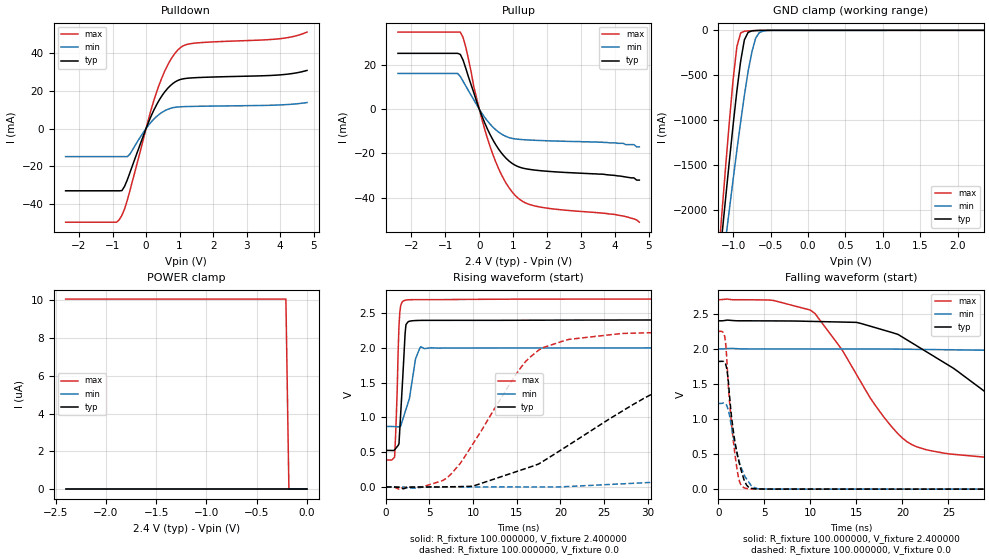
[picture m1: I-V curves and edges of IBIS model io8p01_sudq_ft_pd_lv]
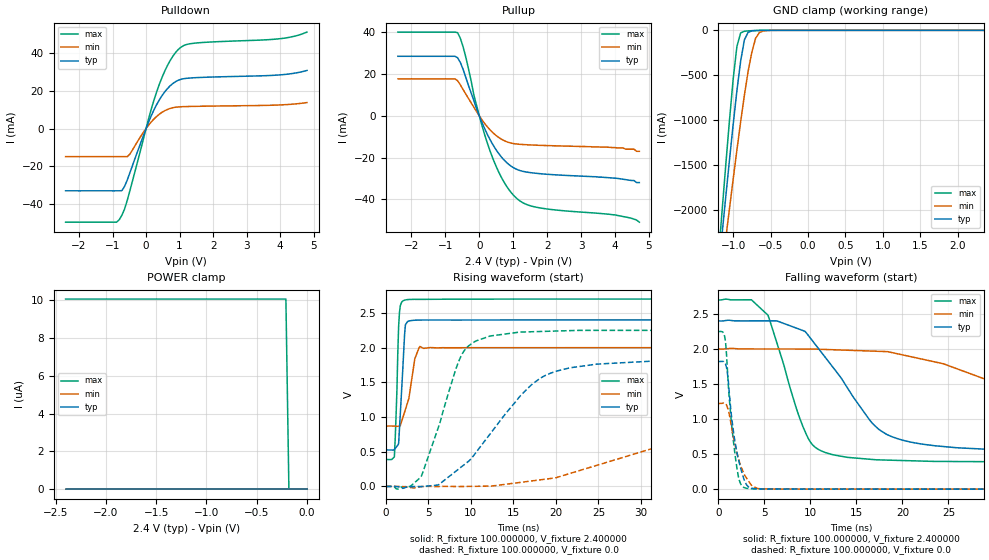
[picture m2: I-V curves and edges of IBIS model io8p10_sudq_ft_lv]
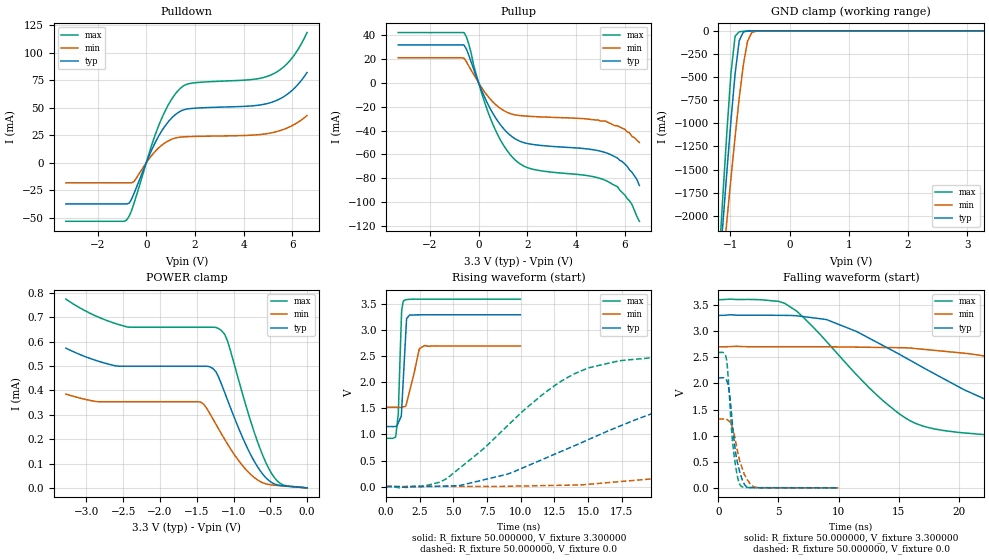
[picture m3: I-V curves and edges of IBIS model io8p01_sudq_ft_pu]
|   stm32f0_440_ufbga64 IBIS Model
[IBIS ver]   4.2
[File name]  stm32f0_440_ufbga64.ibs
[File Rev]   1.0
[Date]   15-5-2013
[Source] Data Created at STMicroelectronics
[Notes]   File originated from ELDO simulations.
[Disclaimer]  This information is for modeling purpose only and is
   not guaranted. The information is subject to change without
   notice.
[Copyright] Copyright 2015 STMicroelectronics Inc.
[Component] stm32f0_440_ufbga64
[Manufacturer] STMicroelectronics
[Package]
| variable   typ   min   max
R_pkg   0.0   NA   NA
L_pkg   0.0H   NA   NA
C_pkg   0.0F   NA   NA
[Pin] signal_name  model_name   R_pin   L_pin   C_pin
B2   VBAT  POWER
A2   PC13  io8p_sudq_tc
A1   PC14  io8p_sudq_tc
B1   PC15  io8p_sudq_tc
C1   PF0   io8p_sudq_ft
D1   PF1   io8p_sudq_ft
E1   NRST  ioreset_tc_v33
E3   PC0   io8p_sudq_ft
E2   PC1   io8p_sudq_ft
F2   PC2   io8p_sudq_ft
G1   PC3   io8p_sudq_ft
F1   VSSA  GND
H1   VDDA  POWER
G2   PA0   io8p_sudq_ft
H2   PA1   io8p_sudq_ft
F3   PA2   io8p_sudq_ft
G3   PA3   io8p_sudq_ft
C2   PF4   io8p_sudq_ft
D2   PF5   io8p_sudq_ft
H3   PA4   io8p_sudq_ft
F4   PA5   io8p_sudq_ft
G4   PA6   io8p_sudq_ft
H4   PA7   io8p_sudq_ft
H5   PC4   io8p_sudq_ft
H6   PC5   io8p_sudq_ft
F5   PB0   io8p_sudq_ft
G5   PB1   io8p_sudq_ft
G6   PB2   io8p_sudq_ft
G7   PB10  io8p_sudq_i2cin_lv_ft
H7   PB11  io8p_sudq_i2cin_lv_ft
D4   VSS   GND
E4   VDD   POWER
H8   PB12  io8p_sudq_ft
G8   PB13  io8p_sudq_ft
F8   PB14  io8p_sudq_ft
F7   PB15  io8p_sudq_ft
F6   PC6   io8p_sudq_ft
E7   PC7   io8p_sudq_ft
E8   PC8   io8p_sudq_ft
D8   PC9   io8p_sudq_ft
D7   PA8   io8p_sudq_ft
C7   PA9   io8p_sudq_ft
C6   PA10  io8p_sudq_ft
C8   PA11  io8p_sudq_ft
B8   PA12  io8p_sudq_ft
A8   PA13  io8p_sudq_ft
D6   PF6   io8p_sudq_i2cin_lv_ft
E6   PF7   io8p_sudq_i2cin_lv_ft
A7   PA14  io8p_sudq_ft
A6   PA15  io8p_sudq_ft
B7   PC10  io8p_sudq_ft
B6   PC11  io8p_sudq_ft
C5   PC12  io8p_sudq_ft
B5   PD2   io8p_sudq_ft
A5   PB3   io8p_sudq_ft
A4   PB4   io8p_sudq_ft
C4   PB5   io8p_sudq_ft
D3   PB6   io8p_sudq_i2cin_lv_ft
C3   PB7   io8p_sudq_i2cin_lv_ft
B4   BOOT0 vpp_test_hv
B3   PB8   io8p_sudq_i2cin_lv_ft
A3   PB9   io8p_sudq_i2cin_lv_ft
D5   VSS   GND
E5   VDD   POWER
[Model Selector] io8p_sudq_ft
io8p01_sudq_ft_pd_lv  "SPEED01 2P0V, PD=40kOhm"
io8p01_sudq_ft_pu_lv  "SPEED01 2P0V, PU=40kOhm"
io8p01_sudq_ft_lv  "SPEED01 2P0V"
io8p10_sudq_ft_pd_lv  "SPEED10 2P0V, PD=40kOhm"
io8p10_sudq_ft_pu_lv  "SPEED10 2P0V, PU=40kOhm"
io8p10_sudq_ft_lv  "SPEED10 2P0V"
io8p11_sudq_ft_pd_lv  "SPEED11 2P0V, PD=40kOhm"
io8p11_sudq_ft_pu_lv  "SPEED11 2P0V, PU=40kOhm"
io8p11_sudq_ft_lv  "SPEED11 2P0V"
io8p01_sudq_ft_pd  "SPEED01, PD=40kOhm"
io8p01_sudq_ft_pu  "SPEED01, PU=40kOhm"
io8p01_sudq_ft  "SPEED01"
io8p10_sudq_ft_pd  "SPEED10, PD=40kOhm"
io8p10_sudq_ft_pu  "SPEED10, PU=40kOhm"
io8p10_sudq_ft  "SPEED10"
io8p11_sudq_ft_pd  "SPEED11, PD=40kOhm"
io8p11_sudq_ft_pu  "SPEED11, PU=40kOhm"
io8p11_sudq_ft  "SPEED11"
[Model Selector] io8p_sudq_i2cin_lv_ft
io8p01_sudq_i2cin_lv_ft_pd_lv  "SPEED01 2P0V, PD=40kOhm"
io8p01_sudq_i2cin_lv_ft_pu_lv  "SPEED01 2P0V, PU=40kOhm"
io8p01_sudq_i2cin_lv_ft_lv  "SPEED01 2P0V"
io8p10_sudq_i2cin_lv_ft_pd_lv  "SPEED10 2P0V, PD=40kOhm"
io8p10_sudq_i2cin_lv_ft_pu_lv  "SPEED10 2P0V, PU=40kOhm"
io8p10_sudq_i2cin_lv_ft_lv  "SPEED10 2P0V"
io8p11_sudq_i2cin_lv_ft_pd_lv  "SPEED11 2P0V, PD=40kOhm"
io8p11_sudq_i2cin_lv_ft_pu_lv  "SPEED11 2P0V, PU=40kOhm"
io8p11_sudq_i2cin_lv_ft_lv  "SPEED11 2P0V"
io8p01_sudq_i2cin_lv_ft_pd  "SPEED01, PD=40kOhm"
io8p01_sudq_i2cin_lv_ft_pu  "SPEED01, PU=40kOhm"
io8p01_sudq_i2cin_lv_ft  "SPEED01"
io8p10_sudq_i2cin_lv_ft_pd  "SPEED10, PD=40kOhm"
io8p10_sudq_i2cin_lv_ft_pu  "SPEED10, PU=40kOhm"
io8p10_sudq_i2cin_lv_ft  "SPEED10"
io8p11_sudq_i2cin_lv_ft_pd  "SPEED11, PD=40kOhm"
io8p11_sudq_i2cin_lv_ft_pu  "SPEED11, PU=40kOhm"
io8p11_sudq_i2cin_lv_ft  "SPEED11"
[Model Selector] io8p_sudq_tc
io8p01_sudq_tc_pd_lv  "SPEED01 2P0V, PD=40kOhm"
io8p01_sudq_tc_pu_lv  "SPEED01 2P0V, PU=40kOhm"
io8p01_sudq_tc_lv  "SPEED01 2P0V"
io8p10_sudq_tc_pd_lv  "SPEED10 2P0V, PD=40kOhm"
io8p10_sudq_tc_pu_lv  "SPEED10 2P0V, PU=40kOhm"
io8p10_sudq_tc_lv  "SPEED10 2P0V"
io8p11_sudq_tc_pd_lv  "SPEED11 2P0V, PD=40kOhm"
io8p11_sudq_tc_pu_lv  "SPEED11 2P0V, PU=40kOhm"
io8p11_sudq_tc_lv  "SPEED11 2P0V"
io8p01_sudq_tc_pd  "SPEED01, PD=40kOhm"
io8p01_sudq_tc_pu  "SPEED01, PU=40kOhm"
io8p01_sudq_tc  "SPEED01"
io8p10_sudq_tc_pd  "SPEED10, PD=40kOhm"
io8p10_sudq_tc_pu  "SPEED10, PU=40kOhm"
io8p10_sudq_tc  "SPEED10"
io8p11_sudq_tc_pd  "SPEED11, PD=40kOhm"
io8p11_sudq_tc_pu  "SPEED11, PU=40kOhm"
io8p11_sudq_tc  "SPEED11"
[Model Selector] ioreset_tc_v33
ioreset_tc_v33_pu_lv  "IORESET 2V + PU=40kOhm"
ioreset_tc_v33_nopu_lv  "IORESET 2V"
ioreset_tc_v33_pu  "IORESET + PU=40kOhm"
ioreset_tc_v33_nopu  "IORESET"
[Model Selector] vpp_test_hv
vpp_test_hv_3p3  "Input Buffer"
vpp_test_hv_2p4  "Input Buffer 2P0V"
| Models and submodels in the file (60): io8p01_sudq_ft_pd_lv (I/O), io8p01_sudq_ft_pu_lv (I/O), io8p01_sudq_ft_lv (I/O), io8p10_sudq_ft_pd_lv (I/O), io8p10_sudq_ft_pu_lv (I/O), io8p10_sudq_ft_lv (I/O), io8p11_sudq_ft_pd_lv (I/O), io8p11_sudq_ft_pu_lv (I/O), io8p11_sudq_ft_lv (I/O), io8p01_sudq_ft_pd (I/O), io8p01_sudq_ft_pu (I/O), io8p01_sudq_ft (I/O), io8p10_sudq_ft_pd (I/O), io8p10_sudq_ft_pu (I/O), io8p10_sudq_ft (I/O), io8p11_sudq_ft_pd (I/O), io8p11_sudq_ft_pu (I/O), io8p11_sudq_ft (I/O), io8p01_sudq_i2cin_lv_ft_pd_lv (I/O), io8p01_sudq_i2cin_lv_ft_pu_lv (I/O), io8p01_sudq_i2cin_lv_ft_lv (I/O), io8p10_sudq_i2cin_lv_ft_pd_lv (I/O), io8p10_sudq_i2cin_lv_ft_pu_lv (I/O), io8p10_sudq_i2cin_lv_ft_lv (I/O), io8p11_sudq_i2cin_lv_ft_pd_lv (I/O), io8p11_sudq_i2cin_lv_ft_pu_lv (I/O), io8p11_sudq_i2cin_lv_ft_lv (I/O), io8p01_sudq_i2cin_lv_ft_pd (I/O), io8p01_sudq_i2cin_lv_ft_pu (I/O), io8p01_sudq_i2cin_lv_ft (I/O), io8p10_sudq_i2cin_lv_ft_pd (I/O), io8p10_sudq_i2cin_lv_ft_pu (I/O), io8p10_sudq_i2cin_lv_ft (I/O), io8p11_sudq_i2cin_lv_ft_pd (I/O), io8p11_sudq_i2cin_lv_ft_pu (I/O), io8p11_sudq_i2cin_lv_ft (I/O), io8p01_sudq_tc_pd_lv (I/O), io8p01_sudq_tc_pu_lv (I/O), io8p01_sudq_tc_lv (I/O), io8p10_sudq_tc_pd_lv (I/O), io8p10_sudq_tc_pu_lv (I/O), io8p10_sudq_tc_lv (I/O), io8p11_sudq_tc_pd_lv (I/O), io8p11_sudq_tc_pu_lv (I/O), io8p11_sudq_tc_lv (I/O), io8p01_sudq_tc_pd (I/O), io8p01_sudq_tc_pu (I/O), io8p01_sudq_tc (I/O), io8p10_sudq_tc_pd (I/O), io8p10_sudq_tc_pu (I/O), io8p10_sudq_tc (I/O), io8p11_sudq_tc_pd (I/O), io8p11_sudq_tc_pu (I/O), io8p11_sudq_tc (I/O), ioreset_tc_v33_pu_lv (I/O_open_drain), ioreset_tc_v33_nopu_lv (I/O_open_drain), ioreset_tc_v33_pu (I/O_open_drain), ioreset_tc_v33_nopu (I/O_open_drain), vpp_test_hv_2p4 (Input), vpp_test_hv_3p3 (Input)
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|   Model io8p01_sudq_ft_pd_lv
[Model]  io8p01_sudq_ft_pd_lv
Model_type I/O
Polarity   Non-Inverting
Enable   Active-Low
Vinl =   0.720000V
Vinh =   1.680000V
Vmeas =  1.200000V
Cref =   50.000000pF
Rref =   100.000000M
Vref =   0.0V
C_comp   1.970100pF   1.887900pF   2.069400pF
[Temperature Range]   25.000000   0.125000k   -40.000000
[Pullup Reference]   2.400000V   2.000000V   2.700000V
[Pulldown Reference]   0.0V   0.0V   0.0V
[POWER Clamp Reference]   2.400000V   2.000000V   2.700000V
[GND Clamp Reference]   0.0V   0.0V   0.0V
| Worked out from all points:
|   slope of the pulldown table from 0 to 0.36 V, typ, clamps not added: 25.5 ohm
|   slope of the pullup table from 0 to 0.36 V, typ, clamps not added: 28.4 ohm
|   GND clamp passes 1 mA (typ) near -0.64 V on its own axis
|   rising waveform, R_fixture 100.000000, V_fixture 2.400000: 20-80 % time 499ps typ, 1.06ns min, 336ps max; typ from 0.525 V to 2.4 V
|   rising waveform, R_fixture 100.000000, V_fixture 0.0: 20-80 % time 14.6ns typ, 43.7ns min, 6.88ns max; typ from 0 V to 1.82 V
|   falling waveform, R_fixture 100.000000, V_fixture 2.400000: 20-80 % time 12.9ns typ, 32.5ns min, 7.07ns max; typ from 2.4 V to 0.525 V
|   falling waveform, R_fixture 100.000000, V_fixture 0.0: 20-80 % time 1.15ns typ, 1.36ns min, 910ps max; typ from 1.82 V to 0 V
[Pulldown]
|Voltage   I(typ)   I(min)   I(max)
-2.4V     -33.16mA   -14.98mA   -49.86mA
-880mV    -33.16mA   -14.98mA   -49.86mA
-800mV    -33.16mA   -14.98mA   -48.55mA
-640mV    -30.75mA   -14.98mA   -42.76mA
-480mV    -23.43mA   -13.57mA   -32.92mA
80mV      3.651mA    1.905mA    5.506mA
400mV     15.37mA    7.665mA    23.73mA
720mV     22.75mA    10.69mA    36.23mA
1.04V     26.18mA    11.57mA    43.27mA
1.52V     27.09mA    11.81mA    45.55mA
4V        28.55mA    12.55mA    47.81mA
4.8V      30.9mA     13.81mA    51.31mA
[Pullup]
|Voltage   I(typ)   I(min)   I(max)
-2.4V     25.2mA     16.13mA    34.79mA
-640mV    25.2mA     16.13mA    34.79mA
-560mV    24.71mA    14.75mA    34.79mA
-400mV    18.51mA    10.48mA    28.09mA
-160mV    7.338mA    4.152mA    10.02mA
80mV      -3.229mA   -1.94mA    -4.736mA
400mV     -13.82mA   -8.081mA   -20.45mA
800mV     -22.31mA   -12.38mA   -33.66mA
1.2V      -26.24mA   -13.65mA   -40.83mA
1.76V     -27.69mA   -14.12mA   -44.07mA
4V        -29.9mA    -15.2mA    -47.5mA
4.72V     -32mA      -17mA      -51mA
[GND_clamp]
|Voltage   I(typ)   I(min)   I(max)
-2.4V     -9.788A    -9.782A    -9.734A
-1.2V     -2.718A    -3.021A    -2.568A
-1.15V    -2.29A     -2.675A    -2.036A
-1.1V     -1.868A    -2.333A    -1.515A
-1.05V    -1.454A    -1.995A    -1.012A
-950mV    -674.5mA   -1.337A    -180.6mA
-900mV    -345.2mA   -1.023A    -29.74mA
-850mV    -106.4mA   -726mA     -10.14mA
-750mV    -6.411mA   -244mA     -4.042mA
-700mV    -2.572mA   -88.62mA   -2.346mA
-600mV    -429.6uA   -7.75mA    -383.5uA
2.35V     59.77uA    46.33uA    66.89uA
[POWER_clamp]
|Voltage   I(typ)   I(min)   I(max)
-2.4V     0A         0A         10.06uA
-210mV    0A         0A         10.06uA
-180mV    0A         0A         0A
0V        0A         0A         0A
[Ramp]
| variable   typ   min   max
dV/dt_r  1.09218/14.55718n   0.73266/43.64565n   1.34874/6.87247n
dV/dt_f  1.12429/12.86053n   0.67801/32.45722n   1.38701/7.06387n
R_load = 100.000000
[Rising Waveform]
R_fixture= 100.000000
V_fixture= 2.400000
V_fixture_min= 2.000000
V_fixture_max= 2.700000
|time   V(typ)   V(min)   V(max)
0s        524.8mV    868.7mV    387.2mV
1.001ns   533mV      867mV      427.7mV
1.301ns   579.7mV    865.4mV    1.395V
1.502ns   618.4mV    864.7mV    2.307V
1.602ns   837.8mV    864.4mV    2.512V
2.102ns   1.961V     1.034V     2.677V
2.302ns   2.331V     1.113V     2.684V
3.403ns   2.39V      1.843V     2.691V
4.004ns   2.392V     2.014V     2.691V
49.85ns   2.399V     1.999V     2.699V
[Rising Waveform]
R_fixture= 100.000000
V_fixture= 0.0
V_fixture_min= 0.0
V_fixture_max= 0.0
|time   V(typ)   V(min)   V(max)
0s        1.768nV    15.89nV    1.355nV
7.007ns   1.867mV    822uV      130.1mV
15.02ns   222.8mV    610.6uV    1.635V
17.52ns   330.7mV    351.7uV    1.966V
27.03ns   1.085V     44.44mV    2.204V
34.53ns   1.55V      90.81mV    2.229V
43.04ns   1.723V     239mV      2.246V
84.08ns   1.82V      945.5mV    2.248V
103.1ns   1.82V      1.111V     2.248V
249.2ns   1.82V      1.221V     2.248V
[Falling Waveform]
R_fixture= 100.000000
V_fixture= 2.400000
V_fixture_min= 2.000000
V_fixture_max= 2.700000
|time   V(typ)   V(min)   V(max)
0s        2.399V     1.999V     2.699V
10.01ns   2.391V     1.998V     2.551V
15.02ns   2.376V     1.997V     1.633V
20.02ns   2.165V     1.994V     725.2mV
29.53ns   1.332V     1.979V     449.6mV
35.04ns   877.6mV    1.964V     425.1mV
42.54ns   673.2mV    1.851V     405.8mV
67.07ns   552.7mV    1.286V     389.2mV
85.59ns   536.1mV    1.035V     387.2mV
249.2ns   524.8mV    868.7mV    387.2mV
[Falling Waveform]
R_fixture= 100.000000
V_fixture= 0.0
V_fixture_min= 0.0
V_fixture_max= 0.0
|time   V(typ)   V(min)   V(max)
0s        1.82V      1.221V     2.248V
700.7ps   1.801V     1.221V     2.178V
800.8ps   1.783V     1.214V     2.095V
1.001ns   1.652V     1.164V     1.701V
1.401ns   1.088V     921.6mV    989mV
1.802ns   687.3mV    646.2mV    513.2mV
2.302ns   364.2mV    381.5mV    115.5mV
2.903ns   104.2mV    178.7mV    14.94mV
4.705ns   1.559mV    3.204mV    789.6uV
49.85ns   1.768nV    15.89nV    1.355nV
|   Model io8p10_sudq_ft_lv
[Model]  io8p10_sudq_ft_lv
Model_type I/O
Polarity   Non-Inverting
Enable   Active-Low
Vinl =   0.720000V
Vinh =   1.680000V
Vmeas =  1.200000V
Cref =   50.000000pF
Rref =   100.000000M
Vref =   0.0V
C_comp   1.970100pF   1.887900pF   2.069400pF
[Temperature Range]   25.000000   0.125000k   -40.000000
[Pullup Reference]   2.400000V   2.000000V   2.700000V
[Pulldown Reference]   0.0V   0.0V   0.0V
[POWER Clamp Reference]   2.400000V   2.000000V   2.700000V
[GND Clamp Reference]   0.0V   0.0V   0.0V
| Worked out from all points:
|   slope of the pulldown table from 0 to 0.36 V, typ, clamps not added: 25.5 ohm
|   slope of the pullup table from 0 to 0.36 V, typ, clamps not added: 28.4 ohm
|   GND clamp passes 1 mA (typ) near -0.64 V on its own axis
|   rising waveform, R_fixture 100.000000, V_fixture 2.400000: 20-80 % time 501ps typ, 1.06ns min, 336ps max; typ from 0.525 V to 2.4 V
|   rising waveform, R_fixture 100.000000, V_fixture 0.0: 20-80 % time 7.32ns typ, 21.7ns min, 3.52ns max; typ from 0 V to 1.82 V
|   falling waveform, R_fixture 100.000000, V_fixture 2.400000: 20-80 % time 6.27ns typ, 18.5ns min, 3.33ns max; typ from 2.4 V to 0.525 V
|   falling waveform, R_fixture 100.000000, V_fixture 0.0: 20-80 % time 1.16ns typ, 1.4ns min, 914ps max; typ from 1.82 V to 0 V
[Pulldown]
|Voltage   I(typ)   I(min)   I(max)
-2.4V     -33.16mA   -14.98mA   -49.86mA
-880mV    -33.16mA   -14.98mA   -49.86mA
-800mV    -33.16mA   -14.98mA   -48.55mA
-640mV    -30.75mA   -14.98mA   -42.76mA
-480mV    -23.43mA   -13.57mA   -32.92mA
80mV      3.651mA    1.905mA    5.506mA
400mV     15.37mA    7.665mA    23.73mA
720mV     22.75mA    10.69mA    36.23mA
1.04V     26.18mA    11.57mA    43.27mA
1.52V     27.09mA    11.81mA    45.55mA
4V        28.55mA    12.55mA    47.81mA
4.8V      30.9mA     13.81mA    51.31mA
[Pullup]
|Voltage   I(typ)   I(min)   I(max)
-2.4V     28.57mA    17.75mA    40.17mA
-720mV    28.57mA    17.75mA    40.17mA
-640mV    27.85mA    16.83mA    39.88mA
-480mV    22.38mA    12.65mA    33.22mA
-80mV     3.427mA    2.066mA    4.957mA
160mV     -6.219mA   -3.715mA   -9.137mA
320mV     -11.51mA   -6.781mA   -16.98mA
720mV     -21mA      -11.8mA    -31.54mA
1.12V     -25.77mA   -13.54mA   -39.82mA
1.76V     -27.69mA   -14.12mA   -44.07mA
4V        -29.9mA    -15.2mA    -47.5mA
4.72V     -32mA      -17mA      -51mA
[GND_clamp]
|Voltage   I(typ)   I(min)   I(max)
-2.4V     -9.788A    -9.782A    -9.734A
-1.2V     -2.718A    -3.02A     -2.568A
-1.15V    -2.29A     -2.675A    -2.036A
-1.1V     -1.868A    -2.333A    -1.515A
-1.05V    -1.454A    -1.995A    -1.012A
-950mV    -674.5mA   -1.337A    -180.5mA
-900mV    -345.2mA   -1.023A    -29.72mA
-850mV    -106.4mA   -726mA     -10.13mA
-750mV    -6.396mA   -244mA     -4.026mA
-700mV    -2.558mA   -88.61mA   -2.329mA
-600mV    -416uA     -7.739mA   -368uA
2.35V     0A         0A         0A
[POWER_clamp]
|Voltage   I(typ)   I(min)   I(max)
-2.4V     0A         0A         10.06uA
-210mV    0A         0A         10.06uA
-180mV    0A         0A         0A
0V        0A         0A         0A
[Ramp]
| variable   typ   min   max
dV/dt_r  1.09308/7.31082n   0.73308/21.71145n   1.34964/3.51759n
dV/dt_f  1.12481/6.26349n   0.67631/18.49686n   1.38754/3.32485n
R_load = 100.000000
[Rising Waveform]
R_fixture= 100.000000
V_fixture= 2.400000
V_fixture_min= 2.000000
V_fixture_max= 2.700000
|time   V(typ)   V(min)   V(max)
0s        525.2mV    870.3mV    387.4mV
1.001ns   533.2mV    868.7mV    426.9mV
1.301ns   579.1mV    867.1mV    1.388V
1.502ns   617.1mV    866.5mV    2.304V
1.702ns   1.054V     877mV      2.604V
2.202ns   2.189V     1.072V     2.684V
2.603ns   2.379V     1.227V     2.693V
3.403ns   2.395V     1.838V     2.696V
4.004ns   2.397V     2.017V     2.696V
49.85ns   2.4V       2V         2.7V
[Rising Waveform]
R_fixture= 100.000000
V_fixture= 0.0
V_fixture_min= 0.0
V_fixture_max= 0.0
|time   V(typ)   V(min)   V(max)
0s        1.81nV     16.19nV    1.388nV
2.803ns   -3.281mV   -14.07mV   -1.578mV
4.204ns   -1.834mV   -2.504mV   153.3mV
8.809ns   274.6mV    -1.375mV   1.87V
12.21ns   748.9mV    4.656mV    2.166V
18.02ns   1.547V     92.84mV    2.232V
24.82ns   1.763V     304.5mV    2.249V
40.24ns   1.817V     861.6mV    2.249V
51.85ns   1.822V     1.107V     2.249V
99.7ns    1.822V     1.223V     2.249V
[Falling Waveform]
R_fixture= 100.000000
V_fixture= 2.400000
V_fixture_min= 2.000000
V_fixture_max= 2.700000
|time   V(typ)   V(min)   V(max)
0s        2.4V       2V         2.7V
3.604ns   2.401V     2V         2.703V
5.405ns   2.402V     2V         2.482V
9.81ns    2.189V     2V         715.2mV
14.01ns   1.448V     1.982V     453.6mV
18.22ns   786.7mV    1.963V     414.6mV
25.83ns   591.3mV    1.722V     393.9mV
36.04ns   545.2mV    1.277V     387.5mV
53.05ns   528.1mV    942.3mV    387.4mV
99.7ns    525.2mV    870.3mV    387.4mV
[Falling Waveform]
R_fixture= 100.000000
V_fixture= 0.0
V_fixture_min= 0.0
V_fixture_max= 0.0
|time   V(typ)   V(min)   V(max)
0s        1.822V     1.223V     2.249V
700.7ps   1.802V     1.222V     2.18V
800.8ps   1.785V     1.215V     2.098V
1.001ns   1.656V     1.165V     1.707V
1.401ns   1.093V     924.2mV    997.1mV
1.902ns   616.8mV    592mV      421.8mV
2.302ns   368.5mV    388.7mV    122.4mV
2.903ns   107.4mV    191.2mV    17.72mV
4.705ns   2.748mV    4.47mV     1.93mV
49.85ns   1.81nV     16.19nV    1.388nV
|   Model io8p01_sudq_ft_pu
[Model]  io8p01_sudq_ft_pu
Model_type I/O
Polarity   Non-Inverting
Enable   Active-Low
Vinl =   0.990000V
Vinh =   2.310000V
Vmeas =  1.650000V
Cref =   50.000000pF
Rref =   100.000000M
Vref =   0.0V
C_comp   1.970900pF   1.892300pF   2.063200pF
[Temperature Range]   25.000000   0.125000k   -40.000000
[Pullup Reference]   3.300000V   2.700000V   3.600000V
[Pulldown Reference]   0.0V   0.0V   0.0V
[POWER Clamp Reference]   3.300000V   2.700000V   3.600000V
[GND Clamp Reference]   0.0V   0.0V   0.0V
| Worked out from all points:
|   slope of the pulldown table from 0 to 0.495 V, typ, clamps not added: 20.9 ohm
|   slope of the pullup table from 0 to 0.495 V, typ, clamps not added: 22.2 ohm
|   GND clamp passes 1 mA (typ) near -0.64 V on its own axis
|   rising waveform, R_fixture 50.000000, V_fixture 3.300000: 20-80 % time 269ps typ, 640ps min, 200ps max; typ from 1.15 V to 3.3 V
|   rising waveform, R_fixture 50.000000, V_fixture 0.0: 20-80 % time 12.6ns typ, 30.5ns min, 7.07ns max; typ from 0.001 V to 2.1 V
|   falling waveform, R_fixture 50.000000, V_fixture 3.300000: 20-80 % time 10.9ns typ, 22.8ns min, 6.89ns max; typ from 3.3 V to 1.15 V
|   falling waveform, R_fixture 50.000000, V_fixture 0.0: 20-80 % time 665ps typ, 860ps min, 543ps max; typ from 2.1 V to 0.001 V
[Pulldown]
|Voltage   I(typ)   I(min)   I(max)
-3.3V     -37.45mA   -18.2mA    -53.24mA
-800mV    -37.45mA   -18.2mA    -51.9mA
-700mV    -36.7mA    -18.2mA    -48.48mA
-500mV    -27.71mA   -17.01mA   -36.65mA
500mV     23.91mA    13.38mA    33.24mA
900mV     37.17mA    19.88mA    52.48mA
1.3V      45.55mA    23.01mA    65.5mA
1.8V      49.29mA    23.83mA    72.18mA
4.4V      51.88mA    25.21mA    75.91mA
5.2V      55.41mA    27.53mA    80.72mA
5.9V      64.2mA     32.82mA    93.01mA
6.6V      82.13mA    42.97mA    118.5mA
[Pullup]
|Voltage   I(typ)   I(min)   I(max)
-3.3V     31.71mA    20.99mA    42.06mA
-600mV    31.71mA    20.58mA    42.06mA
-400mV    22.98mA    13.87mA    32.1mA
0V        90fA       16.1pA     0A
500mV     -22.5mA    -14.16mA   -30.52mA
900mV     -35.28mA   -21.55mA   -48mA
1.4V      -45.55mA   -26.41mA   -62.54mA
2.2V      -51.57mA   -28.22mA   -72.25mA
5.3V      -59.1mA    -33mA      -82.6mA
5.7V      -63mA      -36mA      -87mA
6.2V      -73mA      -42mA      -99mA
6.6V      -86mA      -50mA      -116mA
[GND_clamp]
|Voltage   I(typ)   I(min)   I(max)
-3.3V     -9.525A    -9.501A    -9.513A
-1.2V     -2.719A    -3.023A    -2.568A
-1.13V    -2.122A    -2.541A    -1.826A
-1.06V    -1.537A    -2.065A    -1.111A
-990mV    -975.7mA   -1.599A    -462mA
-920mV    -467.4mA   -1.149A    -59mA
-850mV    -106.6mA   -727.3mA   -10.11mA
-780mV    -13.06mA   -365.4mA   -5.254mA
-710mV    -3.045mA   -114.8mA   -2.635mA
-640mV    -943.2uA   -20.16mA   -905.7uA
-570mV    -199.4uA   -3.959mA   -156.8uA
3.28V     0A         0A         0A
[POWER_clamp]
|Voltage   I(typ)   I(min)   I(max)
-3.28V    574uA      385.1uA    775.2uA
-2.88V    524.3uA    354.9uA    706.9uA
-2.44V    499.6uA    353.9uA    660.7uA
-1.44V    499.6uA    351.4uA    659.6uA
-1.28V    490.1uA    283.2uA    659.6uA
-1.16V    423.2uA    219.6uA    645uA
-1.08V    359.8uA    179.3uA    602.1uA
-800mV    156.6uA    65uA       306.5uA
-640mV    71.59uA    26.48uA    162uA
-520mV    30.4uA     13.8uA     79.2uA
-360mV    9.635uA    8.674uA    17.24uA
0V        0A         0A         0A
[Ramp]
| variable   typ   min   max
dV/dt_r  1.26228/12.61797n   0.78952/30.42228n   1.55421/7.05616n
dV/dt_f  1.28868/10.87235n   0.70572/22.79880n   1.60392/6.88172n
R_load = 50.000000
[Rising Waveform]
R_fixture= 50.000000
V_fixture= 3.300000
V_fixture_min= 2.700000
V_fixture_max= 3.600000
|time   V(typ)   V(min)   V(max)
0s        1.152V     1.524V     926.8mV
720.7ps   1.154V     1.523V     980.8mV
900.9ps   1.224V     1.522V     1.396V
1.141ns   1.424V     1.525V     3.317V
1.261ns   2.003V     1.53V      3.557V
1.522ns   3.23V      1.607V     3.591V
1.762ns   3.296V     1.853V     3.596V
2.462ns   3.299V     2.646V     3.599V
2.863ns   3.3V       2.709V     3.599V
9.97ns    3.3V       2.7V       3.6V
[Rising Waveform]
R_fixture= 50.000000
V_fixture= 0.0
V_fixture_min= 0.0
V_fixture_max= 0.0
|time   V(typ)   V(min)   V(max)
0s        1.102mV    1.228mV    1.054mV
4.505ns   9.75mV     3.271mV    154.5mV
9.009ns   238.2mV    4.996mV    1.167V
14.01ns   786.9mV    29.27mV    2.169V
22.02ns   1.592V     198mV      2.526V
27.53ns   1.886V     332.4mV    2.56V
38.54ns   2.055V     659.5mV    2.588V
55.56ns   2.101V     1.056V     2.592V
75.08ns   2.104V     1.241V     2.591V
249.2ns   2.105V     1.317V     2.592V
[Falling Waveform]
R_fixture= 50.000000
V_fixture= 3.300000
V_fixture_min= 2.700000
V_fixture_max= 3.600000
|time   V(typ)   V(min)   V(max)
0s        3.3V       2.7V       3.6V
5.506ns   3.3V       2.701V     3.532V
9.009ns   3.22V      2.7V       2.799V
13.01ns   2.808V     2.688V     1.815V
16.02ns   2.435V     2.675V     1.278V
22.52ns   1.666V     2.512V     1.015V
27.53ns   1.377V     2.339V     970.5mV
41.54ns   1.204V     1.849V     936.2mV
69.57ns   1.158V     1.588V     927mV
249.2ns   1.152V     1.524V     926.8mV
[Falling Waveform]
R_fixture= 50.000000
V_fixture= 0.0
V_fixture_min= 0.0
V_fixture_max= 0.0
|time   V(typ)   V(min)   V(max)
0s        2.105V     1.317V     2.592V
660.7ps   2.063V     1.316V     2.467V
900.9ps   1.841V     1.274V     1.796V
1.141ns   1.274V     1.166V     952.7mV
1.261ns   976.7mV    1.075V     695mV
1.602ns   464.4mV    685.9mV    193.9mV
1.862ns   238mV      452mV      38.35mV
2.282ns   34.99mV    204mV      8.533mV
3.103ns   3.072mV    11.74mV    4.654mV
9.97ns    1.102mV    1.228mV    1.054mV
